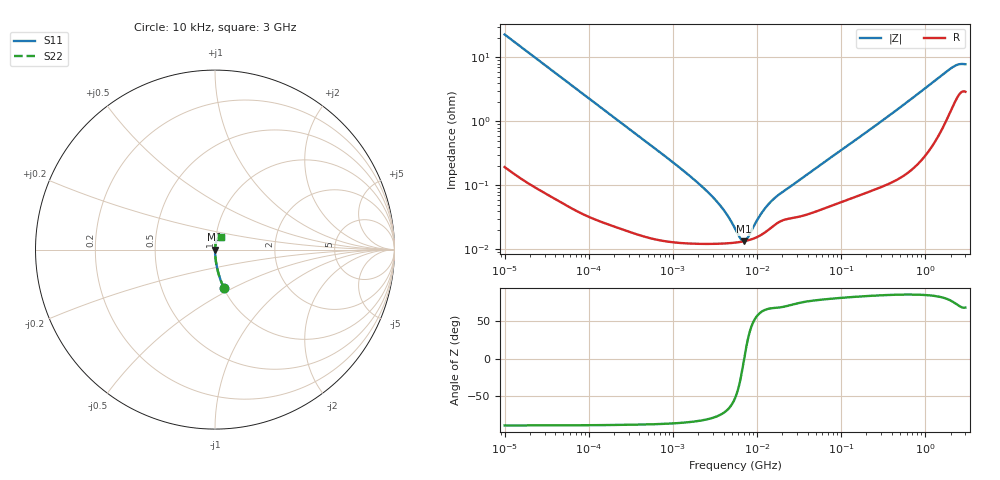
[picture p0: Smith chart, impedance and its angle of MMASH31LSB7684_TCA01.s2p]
! MMASH31LSB7684_TCA01  S-PARAMETER MODEL  ( Standard Model )
! Model Generated by TAIYO YUDEN Corporation (http://www.ty-top.com)
! Version 1.0
! TAIYO YUDEN Control No. 220601
! Copyright(c) 2022 TAIYO YUDEN CO.,LTD. All Rights Reserved.
! Product Description (link to TY-COMPAS)
! https://ds.yuden.co.jp/TYCOMPAS/or/detail?pn=MMASH31LSB7684KTCA01&u=M
! Products Name : Multilayer Ceramic Capacitors
! Characteristics :
!  Capacitance : 0.68 [uF] , Rated Voltage : 100 [V] , TCC : X7R
!  Case Size : 3.2 x 1.6 / 0.126 x 0.063 [mm/inch] , Thickness : 1.6 / 0.063 [mm/inch]
!  (Conditions: Temperature = 25 [degC] , DC Bias Voltage = 0 [V])
! External Node Assignments :
!  1  o---| |---o  2
! GND o---------o GND
! Frequency Range : 10kHz  -  3GHz  [ 401 STEP ]
# MHZ S RI R 50
! Freq[MHz].  S11 Real  S11 Imag  S21 Real  S21 Imag  S12 Real  S12 Imag  S22 Real  S22 Imag
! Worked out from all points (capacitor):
!   401 points, 10 kHz to 3 GHz, reference 50 ohm
!   read as one part in series: C = 698 nF near 10.65 kHz
!   lowest |Z| = 13.4 mohm at 7.049 MHz (marker M1)
!   series resonance near 7.05 MHz, so ESL is about 730 pH
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0.01  0.051 -0.2158  0.949 0.2158  0.949 0.2158  0.051 -0.2158
0.016047  0.021 -0.1391  0.979 0.1391  0.979 0.1391  0.021 -0.1391
0.02575  0.00867 -0.088  0.9913 0.088  0.9913 0.088  0.00867 -0.088
0.082683  0.00114 -0.0278  0.9989 0.0278  0.9989 0.0278  0.00114 -0.0278
0.683653  0.000151 -0.00338  0.9998 0.00338  0.9998 0.00338  0.000151 -0.00338
1.652853  0.000125 -0.00134  0.9999 0.00134  0.9999 0.00134  0.000125 -0.00134
2.824956  0.000122 -0.000696  0.9999 0.000696  0.9999 0.000696  0.000122 -0.000696
4.124064  0.000124 -0.000374  0.9999 0.000374  0.9999 0.000374  0.000124 -0.000374
4.828246  0.000125 -0.000258  0.9999 0.000258  0.9999 0.000258  0.000125 -0.000258
5.477226  0.000127 -0.00017  0.9999 0.00017  0.9999 0.00017  0.000127 -0.00017
6.41246  0.000131 -6.33e-05  0.9999 6.33e-05  0.9999 6.33e-05  0.000131 -6.33e-05
7.048603  0.000134 -1.26e-07  0.9999 1.26e-07  0.9999 1.26e-07  0.000134 -1.26e-07
7.747855  0.000138 6.31e-05  0.9999 -6.31e-05  0.9999 -6.31e-05  0.000138 6.31e-05
9.97066  0.000155 0.000236  0.9998 -0.000236  0.9998 -0.000236  0.000155 0.000236
11.31085  0.000169 0.000326  0.9998 -0.000326  0.9998 -0.000326  0.000169 0.000326
14.55585  0.000216 0.00051  0.9998 -0.00051  0.9998 -0.00051  0.000216 0.00051
18.15044  0.000266 0.000664  0.9997 -0.000664  0.9997 -0.000664  0.000266 0.000664
45.28751  0.000374 0.00165  0.9996 -0.00165  0.9996 -0.00165  0.000374 0.00165
374.4521  0.00122 0.0123  0.9988 -0.0123  0.9988 -0.0123  0.00122 0.0123
1991.2  0.018 0.0629  0.982 -0.0629  0.982 -0.0629  0.018 0.0629
2482.93  0.0297 0.0694  0.9703 -0.0694  0.9703 -0.0694  0.0297 0.0694
3000  0.033 0.0682  0.967 -0.0682  0.967 -0.0682  0.033 0.0682
